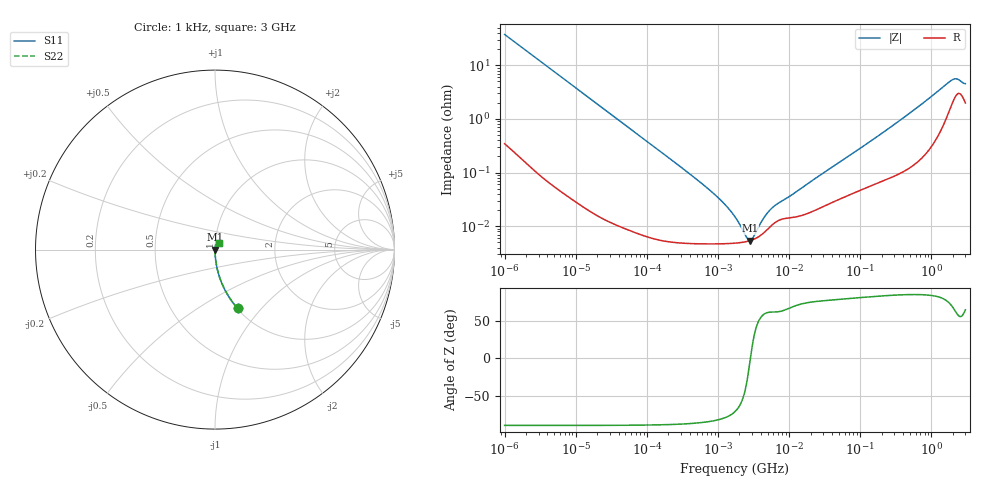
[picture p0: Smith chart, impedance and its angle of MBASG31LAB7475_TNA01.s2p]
! MBASG31LAB7475_TNA01  S-PARAMETER MODEL  ( Standard Model )
! Model Generated by TAIYO YUDEN Corporation (http://www.ty-top.com)
! Version 1.0
! TAIYO YUDEN Control No. 220601
! Copyright(c) 2012 TAIYO YUDEN CO.,LTD. All Rights Reserved.
! Product Description (link to TY-COMPAS)
! https://ds.yuden.co.jp/TYCOMPAS/or/detail?pn=MBASG31LAB7475KTNA01&u=M
! Products Name : Multilayer Ceramic Capacitors
! Characteristics :
!  Capacitance : 4.7 [uF] , Rated Voltage : 35 [V] , TCC : X7R
!  Case Size : 3.2 x 1.6 / 0.126 x 0.063 [mm/inch] , Thickness : 1.6 / 0.063 [mm/inch]
!  (Conditions: Temperature = 25 [degC] , DC Bias Voltage = 0 [V])
! External Node Assignments :
!  1  o---| |---o  2
! GND o---------o GND
! Frequency Range : 1kHz  -  3GHz  [ 401 STEP ]
# MHZ S RI R 50
! Freq[MHz].  S11 Real  S11 Imag  S21 Real  S21 Imag  S12 Real  S12 Imag  S22 Real  S22 Imag
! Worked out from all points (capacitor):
!   401 points, 1 kHz to 3 GHz, reference 50 ohm
!   read as one part in series: C = 4.22 uF near 1.077 kHz
!   lowest |Z| = 5.39 mohm at 2.812 MHz (marker M1)
!   series resonance near 2.855 MHz, so ESL is about 740 pH
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0.001  0.1265 -0.3279  0.8735 0.3279  0.8735 0.3279  0.1265 -0.3279
0.001685  0.0495 -0.2127  0.9505 0.2127  0.9505 0.2127  0.0495 -0.2127
0.00306  0.016 -0.1217  0.984 0.1217  0.984 0.1217  0.016 -0.1217
0.005768  0.00478 -0.0655  0.9952 0.0655  0.9952 0.0655  0.00478 -0.0655
0.01216  0.00122 -0.0313  0.9988 0.0313  0.9988 0.0313  0.00122 -0.0313
0.147855  6.19e-05 -0.00259  0.9999 0.00259  0.9999 0.00259  6.19e-05 -0.00259
0.43594  4.8e-05 -0.000863  1 0.000863  1 0.000863  4.8e-05 -0.000863
0.821683  4.69e-05 -0.000431  1 0.000431  1 0.000431  4.69e-05 -0.000431
1.285341  4.73e-05 -0.00024  1 0.00024  1 0.00024  4.73e-05 -0.00024
1.732051  4.83e-05 -0.000142  1 0.000142  1 0.000142  4.83e-05 -0.000142
2.010629  4.92e-05 -9.77e-05  1 9.77e-05  1 9.77e-05  4.92e-05 -9.77e-05
2.166294  4.99e-05 -7.64e-05  1 7.64e-05  1 7.64e-05  4.99e-05 -7.64e-05
2.812335  5.38e-05 -4.1e-06  0.9999 4.1e-06  0.9999 4.1e-06  5.38e-05 -4.1e-06
3.651041  6.26e-05 6.85e-05  0.9999 -6.85e-05  0.9999 -6.85e-05  6.26e-05 6.85e-05
3.93371  6.69e-05 8.97e-05  0.9999 -8.97e-05  0.9999 -8.97e-05  6.69e-05 8.97e-05
5.106836  9.06e-05 0.000163  0.9999 -0.000163  0.9999 -0.000163  9.06e-05 0.000163
6.153411  0.000114 0.000208  0.9999 -0.000208  0.9999 -0.000208  0.000114 0.000208
21.06097  0.000187 0.000684  0.9998 -0.000684  0.9998 -0.000684  0.000187 0.000684
256.0921  0.000826 0.00673  0.9992 -0.00673  0.9992 -0.00673  0.000826 0.00673
1917.819  0.0201 0.0477  0.9799 -0.0477  0.9799 -0.0477  0.0201 0.0477
2226.275  0.029 0.0463  0.971 -0.0463  0.971 -0.0463  0.029 0.0463
3000  0.021 0.0394  0.979 -0.0394  0.979 -0.0394  0.021 0.0394
